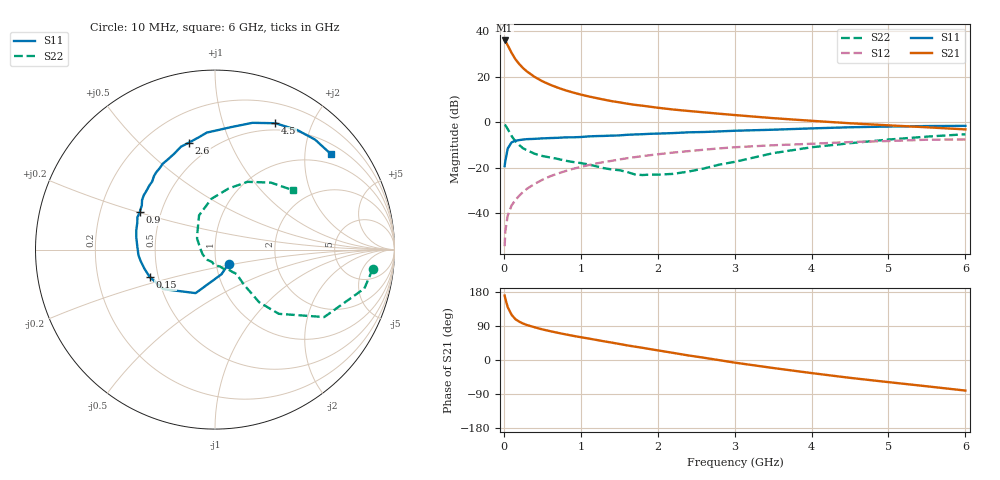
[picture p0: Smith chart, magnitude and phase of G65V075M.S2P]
! SIEMENS Small Signal Semiconductors
! BFG193
! Si NPN RF Bipolar Junction Transistor in SOT223
! VCE = 5 V  IC = 75 mA
! Common Emitter S-Parameters:  August  1996
# GHz  S  MA  R  50
!  f  S11  S21  S12  S22
! GHz  MAG  ANG  MAG  ANG  MAG  ANG  MAG  ANG
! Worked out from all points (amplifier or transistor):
!   36 points, 10 MHz to 6 GHz, reference 50 ohm
!   highest |S21| = 36.0 dB at 10 MHz (marker M1)
!   |S21| within 3 dB of that: start of sweep to 63.68 MHz
!   unconditionally stable (mu >= 1): 344 MHz to 2.312 GHz
!   at 250 MHz: K = 0.96, MSG = 27.2 dB, |S12| = -30.6 dB
!   at 1.4 GHz: K = 1.05, MAG = 11.7 dB, |S12| = -16.9 dB
!   at 6 GHz: K = 0.90, MSG = 2.2 dB, |S12| = -7.5 dB
!   S11 on the Smith chart (normalised r, x): 10 MHz: 1.15, -0.18; 150 MHz: 0.45, -0.16; 900 MHz: 0.38, +0.20; 2.6 GHz: 0.37, +0.72; 4.5 GHz: 0.42, +1.50; 6 GHz: 0.74, +2.62
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0.01  0.1092 -45.6  63.08 170.0  0.0019 84.3  0.8854 -7.0
0.02  0.1422 -75.3  60.4 161.6  0.0041 77.6  0.8599 -14.6
0.05  0.2653 -114.0  49.58 139.5  0.0089 71.7  0.7154 -31.7
0.1  0.362 -142.5  33.84 119.6  0.0149 68.0  0.5043 -45.2
0.15  0.3947 -157.4  24.48 107.7  0.0196 68.2  0.383 -50.0
0.2  0.4076 -165.0  19.16 101.2  0.0244 70.6  0.317 -50.2
0.25  0.419 -171.2  15.55 96.2  0.0296 70.6  0.269 -50.4
0.3  0.4276 -175.8  13.14 92.3  0.0346 71.7  0.2435 -50.3
0.4  0.4337 177.3  9.978 86.4  0.0445 71.4  0.2045 -49.3
0.5  0.4443 170.9  8.011 80.8  0.0546 70.0  0.1824 -48.7
0.6  0.4517 166.2  6.729 76.2  0.0651 69.0  0.1694 -50.0
0.7  0.4574 161.3  5.792 71.8  0.0749 67.6  0.1573 -52.2
0.9  0.469 153.3  4.523 63.8  0.0954 63.8  0.1344 -55.7
1.1  0.4909 145.9  3.72 56.7  0.1146 60.3  0.1188 -65.2
1.3  0.5034 139.2  3.161 49.4  0.1341 56.2  0.0984 -73.5
1.6  0.5328 129.6  2.579 38.7  0.1625 49.2  0.0813 -95.4
2.2  0.5807 113.0  1.916 18.8  0.2166 35.6  0.0737 -158.9
2.6  0.6135 103.6  1.66 6.0  0.2502 26.8  0.0968 159.6
3.5  0.6891 82.3  1.237 -21.1  0.3138 4.1  0.2103 115.0
4.5  0.7801 64.5  0.955 -47.1  0.3692 -16.1  0.3479 77.6
5.5  0.8285 47.7  0.779 -69.4  0.4155 -39.6  0.486 50.2
6  0.8371 39.3  0.7 -80.7  0.421 -53.2  0.5472 37.1
